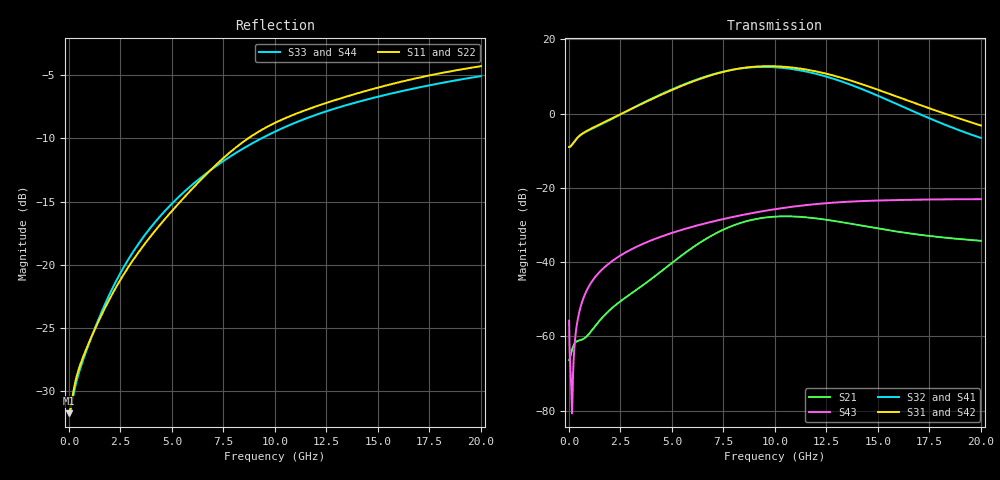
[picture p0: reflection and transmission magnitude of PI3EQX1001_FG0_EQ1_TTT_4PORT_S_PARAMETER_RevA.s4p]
! NPort=4 DATA=2000 NOISE=0 GROUPDELAY=0 COMPLEX_DATAFORMAT=POLAR
! NumOfBlock=1 NumOfParam=0
! .MODEL Smodel S TSTONEFILE=PI3EQX1001_FG0_EQ1_TTT_4PORT_S_PARAMETER_RevA.s4p TYPE=S
!  -- The above .MODEL line can be used for the S element in the netlist.
! The s parameter is extracted from the linear redriver, it is not bi-directional; only s(4,1)s(4,2) and s(3,1)s(3,2)
! should be the insertion loss
!Port definition:
!Port1 = input+
!Port2 = input¨C
!Port3 = output+
!Port4 = output-
# Hz S MA R  50
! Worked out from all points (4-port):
!   2000 points, 10 MHz to 20 GHz, reference 50 ohm
!   strongest paths, dB at 10 MHz, 5.01 GHz, 10.01 GHz, 15.01 GHz, 20 GHz:
!     S31: -9.0, 6.4, 12.7, 6.4, -3.2
!     S42: -9.0, 6.3, 12.7, 6.4, -3.2
!     S32: -9.0, 6.5, 12.5, 4.8, -6.6
!     S41: -9.0, 6.5, 12.4, 4.7, -6.6
!     S43: -55.8, -32.1, -25.8, -23.4, -23.1
!     S21: -66.4, -40.2, -27.8, -31.0, -34.3
!   lowest |S11| = -31.7 dB at 10 MHz (marker M1), VSWR 1.05, Z = 47.5 - j0.063 ohm
!   |S11| at or under -10 dB: start of sweep to 8.702 GHz
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1e7  0.0259 -178.5  0.0004902 2.7  3.669e-05 -0.2  4.787e-05 -0.1
     0.000479 2.9  0.02597 -178.7  4.577e-05 -0.2  5.994e-05 -0.1
     0.3547 0.3  0.3547 -179.6  0.02616 178.4  0.001616 -59.1
     0.3545 -179.6  0.3546 0.4  0.001626 -59.0  0.02613 178.4
6.32e9  0.2134 -104.5  0.0173 98.7  2.284e-05 -30.9  3.268e-05 -29.3
        0.01795 97.0  0.2118 -104.4  2.992e-05 -26.4  4.169e-05 -24.5
        2.902 -48.0  2.945 135.6  0.2184 -111.1  0.03158 61.0
        2.929 135.5  2.895 -48.0  0.03159 61.0  0.2183 -111.1
8.54e9  0.3096 -107.7  0.03396 61.7  2.02e-05 -28.3  3.157e-05 -30.9
        0.035 60.4  0.3076 -107.8  2.951e-05 -25.5  3.915e-05 -24.9
        4.144 -109.1  4.115 74.9  0.2909 -113.6  0.04382 48.4
        4.087 74.9  4.136 -109.1  0.04373 48.2  0.2907 -113.6
1.067e10  0.3852 -114.0  0.04009 22.1  2.184e-05 -23.2  3.358e-05 -40.0
          0.04127 21.0  0.3824 -114.1  3.191e-05 -33.8  4.004e-05 -24.9
          4.213 -173.4  4.036 11.2  0.3557 -117.2  0.05501 34.1
          4.005 11.4  4.205 -173.3  0.05479 34.0  0.3555 -117.1
1.327e10  0.4572 -119.5  0.03332 -12.0  2.852e-05 -37.7  3.111e-05 -63.8
          0.03435 -13.0  0.4534 -119.6  2.929e-05 -56.0  4.544e-05 -35.3
          3.011 114.3  2.686 -59.7  0.4233 -121.7  0.06448 15.5
          2.663 -59.4  3.004 114.3  0.06429 15.6  0.4233 -121.7
1.578e10  0.5212 -124.0  0.02525 -28.0  2.834e-05 -69.6  2.285e-05 -93.8
          0.02613 -29.1  0.5168 -124.0  2.051e-05 -82.9  4.272e-05 -57.3
          1.749 58.0  1.397 -112.4  0.4784 -125.5  0.06836 -0.6
          1.384 -112.0  1.744 58.1  0.06827 -0.5  0.478 -125.5
2e10  0.6101 -131.1  0.01869 -37.3  1.495e-05 -147.8  1.299e-05 152.2
      0.01934 -38.9  0.6047 -131.2  8.988e-06 139.0  1.791e-05 -96.9
      0.6914 -9.6  0.4698 -162.5  0.5572 -131.2  0.07031 -23.8
      0.4666 -161.5  0.6888 -9.5  0.07027 -23.8  0.5571 -131.1
